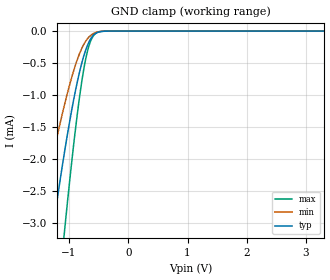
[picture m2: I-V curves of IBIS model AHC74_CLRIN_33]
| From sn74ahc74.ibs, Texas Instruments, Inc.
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[Model]   AHC74_CLRIN_33
Model_type  Input
Vinl = 0.9
Vinh = 2.1
| variable   typ   min   max
C_comp   0.66pF   0.58pF   0.75pF
[Temperature Range]   40   100   -40
| Ambient temperature   25   85   -40
[Voltage range]   3.3   3   3.6
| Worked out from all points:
|   GND clamp passes 1 mA (typ) near -0.91 V on its own axis
[GND Clamp]
| AHC74_CLRIN_33
|   Voltage   I(typ)   I(min)   I(max)
-3.3V     -21.05mA   -13.78mA   -28.64mA
-1.52V    -4.845mA   -3.097mA   -7.647mA
-1.28V    -3.152mA   -1.983mA   -5.117mA
-1.1V     -2.026mA   -1.24mA    -3.347mA
-1.07V    -1.853mA   -1.126mA   -3.066mA
-905mV    -992.8uA   -568.6uA   -1.638mA
-835mV    -688.4uA   -381uA     -1.115mA
-770mV    -449.4uA   -241.7uA   -699.2uA
-675mV    -193uA     -104uA     -265.9uA
-575mV    -52.68uA   -32.06uA   -58.42uA
-375mV    -1.402uA   -1.027uA   -717.1nA
3.3V      3.885nA    645.3pA    18.64nA
